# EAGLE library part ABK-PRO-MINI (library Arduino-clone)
ABK Pro-Mini Arduino Clone
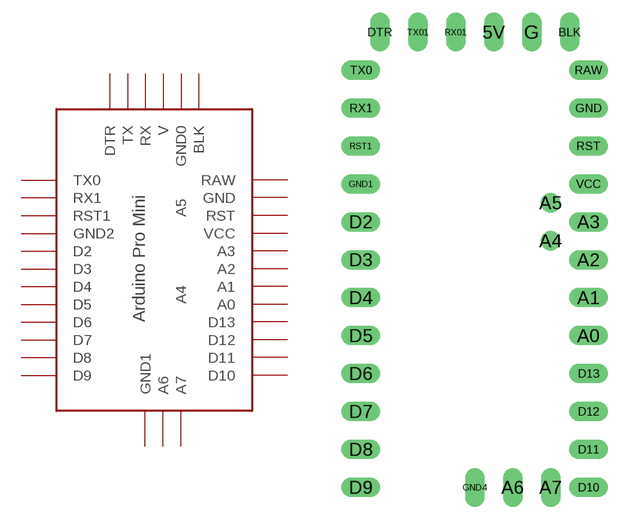
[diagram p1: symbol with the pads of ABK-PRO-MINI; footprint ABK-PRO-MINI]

Designator prefix -

## ABK-PRO-MINI  [ABK-PRO-MINI]
5V  V
A0  A3
A1  A2
A2  A1
A3  A0
A4  A4
A5  A5
A6  A6
A7  A7
BLK  BLK
D2  D2
D3  D3
D4  D4
D5  D5
D6  D6
D7  D7
D8  D8
D9  D9
D10  D10
D11  D11
D12  D12
D13  D13
DTR  DTR
G  GND0
GND  GND
GND1  GND2
GND4  GND1
RAW  RAW
RST  RST
RST1  RST1
RX01  RX
RX1  RX1
TX0  TX0
TX01  TX
VCC  VCC

## Footprint ABK-PRO-MINI (pad centres in mm)
ABK-PRO-MINI
drill 0.8 long: 5V 3.81,8.89; A0 10.16,-11.43; A1 10.16,-8.89; A2 10.16,-6.35; A3 10.16,-3.81; A6 5.08,-21.59; A7 7.62,-21.59; BLK 8.89,8.89; D2 -5.08,-3.81; D3 -5.08,-6.35; D4 -5.08,-8.89; D5 -5.08,-11.43; D6 -5.08,-13.97; D7 -5.08,-16.51; D8 -5.08,-19.05; D9 -5.08,-21.59; D10 10.16,-21.59; D11 10.16,-19.05; D12 10.16,-16.51; D13 10.16,-13.97; DTR -3.81,8.89; G 6.35,8.89; GND 10.16,3.81; GND1 -5.08,-1.27; GND4 2.54,-21.59; RAW 10.16,6.35; RST 10.16,1.27; RST1 -5.08,1.27; RX01 1.27,8.89; RX1 -5.08,3.81; TX0 -5.08,6.35; TX01 -1.27,8.89; VCC 10.16,-1.27
drill 0.8: A4 7.62,-5.08; A5 7.62,-2.54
